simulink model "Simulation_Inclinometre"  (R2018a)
settings: Solver=FixedStepAuto  StartTime=0.0  StopTime=10  FixedStep=0.01  RelTol=1e-3
undefined symbols (not defined in the file): sigbuilder_block
libraries: aerolibconvert2 x1, simulink x1

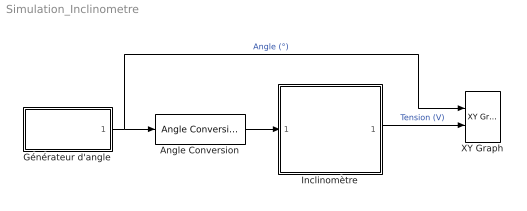
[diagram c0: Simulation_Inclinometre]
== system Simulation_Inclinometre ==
  Angle Conversion : aerolibconvert2/Angle Conversion  IU=deg  OU=rad
  Générateur d'angle : Subsystem  Tag=STV Subsys  LoadFcn=sigbuilder_block('load');  StartFcn=sigbuilder_block('start');  StopFcn=sigbuilder_block('stop');  ClipboardFcn=sigbuilder_block('clipboard');  mask(Sigbuilder block){tuvar=[0:10]}
      mask help: Simulink:masks:SigbuilderBlock_MD
      mask init:
      | if ~strcmp(get_param(bdroot(gcbh),'SimulationStatus'),'stopped') tuvar = sigbuilder_block('maskInit'); end
  Inclinomètre : Subsystem
  XY Graph : simulink/Sinks/XY Graph  xmin=-90  xmax=+90  ymin=1  ymax=2  st=-1
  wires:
  Inclinomètre/1(Tension) -> XY Graph/2  "Tension (V)"
  Angle Conversion/1 -> Inclinomètre/1(Angle)
  Générateur d'angle/1(Signal 1) -> XY Graph/1, Angle Conversion/1  "Angle (°)"

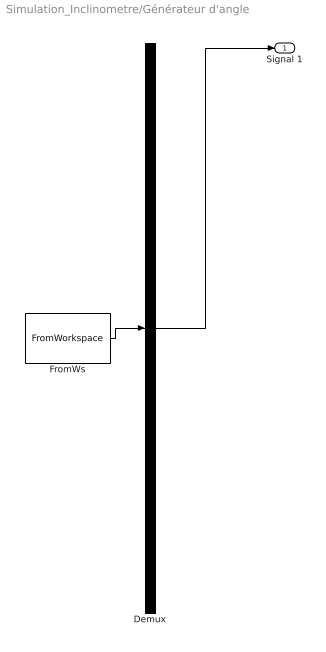
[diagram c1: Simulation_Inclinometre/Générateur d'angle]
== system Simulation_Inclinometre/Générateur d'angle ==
  Demux : Demux  Tag=STV Demux  Outputs=1
  FromWs : FromWorkspace  Tag=STV FromWs  VariableName=tuvar  SampleTime=0
  Signal 1 : Outport  Tag=STV Outport
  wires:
  Demux/1 -> Signal 1/1
  FromWs/1 -> Demux/1

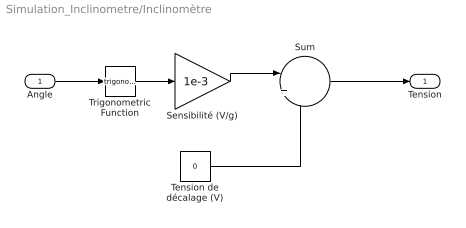
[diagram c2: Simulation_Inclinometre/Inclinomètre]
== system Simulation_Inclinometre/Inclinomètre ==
  Angle : Inport
  Sensibilité (V/g) : Gain  Gain=1e-3
  Sum : Sum  Inputs=|++
  Tension de décalage (V) : Constant  Value=0
  Trigonometric Function : Trigonometry
  Tension : Outport
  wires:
  Tension de décalage (V)/1 -> Sum/2
  Sum/1 -> Tension/1
  Sensibilité (V/g)/1 -> Sum/1
  Trigonometric Function/1 -> Sensibilité (V/g)/1
  Angle/1 -> Trigonometric Function/1
